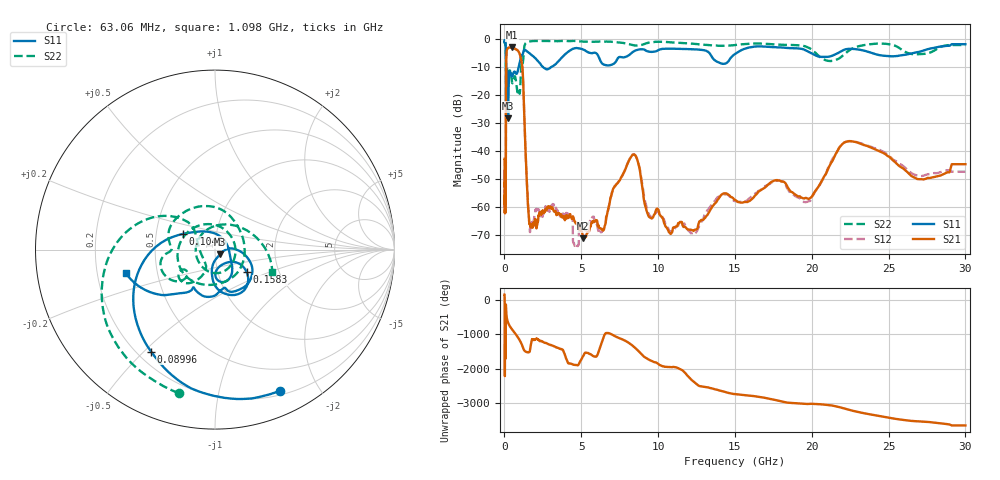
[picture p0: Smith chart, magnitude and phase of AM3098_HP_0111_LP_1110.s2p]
! Date/Time: Thu, Feb 28, 2019 8:39 AM
! Network Analyzer: Agilent Technologies E8364B Rev: A.07.50.67
! Sweep from 0.010 to 30.000 GHz, 1601 Points, Sweep Type: LOG
! Power Supply: 5.022 V, 0.002 A
# Hz S DB R 50
!freq MagS11 AngS11 MagS21 AngS21 MagS12 AngS12 MagS22 AngS22
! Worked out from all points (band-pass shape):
!   1601 points, 10 MHz to 30 GHz, reference 50 ohm
!   highest |S21| = -2.79 dB at 488.2 MHz (marker M1); lowest = -71.1 dB at 5.128 GHz (marker M2)
!   |S21| within 3 dB of the highest: 122.4 MHz to 1.028 GHz (905.7 MHz wide, 157 % of centre)
!   lowest |S11| = -28.2 dB at 238.7 MHz (marker M3), VSWR 1.08, Z = 52.9 - j2.73 ohm
!   |S11| at or under -10 dB: 102.2 MHz to 922.3 MHz (820.1 MHz wide, 160 % of centre); 2.53 GHz to 3.003 GHz (473.2 MHz wide, 17.1 % of centre)
!   |S22| runs from -21.9 to -0.5 dB; largest |S21 - S12| = 0.0094
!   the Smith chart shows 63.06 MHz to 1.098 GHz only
!   S11 on the Smith chart (normalised r, x): 63.06 MHz: 0.24, -1.53; 89.96 MHz: 0.25, -0.53; 104.5 MHz: 0.69, +0.13; 158.3 MHz: 1.37, -0.36; 1.098 GHz: 0.33, -0.12
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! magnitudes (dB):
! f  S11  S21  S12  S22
! 10 MHz  -0.4  -42.7  -46.5  -0.6
! 38.04 MHz  -0.4  -59.6  -61.0  -1.0
! 63.06 MHz  -1.2  -52.9  -53.7  -1.7
! 89.96 MHz  -3.5  -46.6  -46.3  -3.8
! 104.5 MHz  -14.1  -15.7  -15.7  -18.9
! 144.7 MHz  -19.7  -4.0  -4.0  -14.0
! 158.3 MHz  -13.3  -3.7  -3.7  -12.0
! 238.7 MHz  -28.2  -3.0  -3.0  -12.0
! 311.2 MHz  -12.8  -2.9  -2.8  -11.4
! 488.2 MHz  -13.1  -2.8  -2.8  -15.2
! 550.5 MHz  -12.5  -3.0  -2.9  -15.2
! 1.098 GHz  -5.8  -7.6  -7.6  -9.3
! 1.614 GHz  -4.8  -65.4  -65.0  -0.8
! 2.084 GHz  -7.1  -67.6  -60.8  -0.5
! 5.128 GHz  -3.6  -71.1  -66.9  -0.8
! 6.36 GHz  -8.6  -68.1  -68.5  -0.8
! 7.926 GHz  -6.1  -45.6  -45.4  -1.4
! 12.07 GHz  -3.5  -68.0  -68.4  -1.4
! 14.09 GHz  -8.6  -55.7  -55.7  -2.3
! 19.7 GHz  -4.2  -56.8  -58.1  -2.7
! 22.56 GHz  -3.3  -36.4  -36.4  -3.5
! 30 GHz  -1.7  -44.6  -47.3  -2.0
